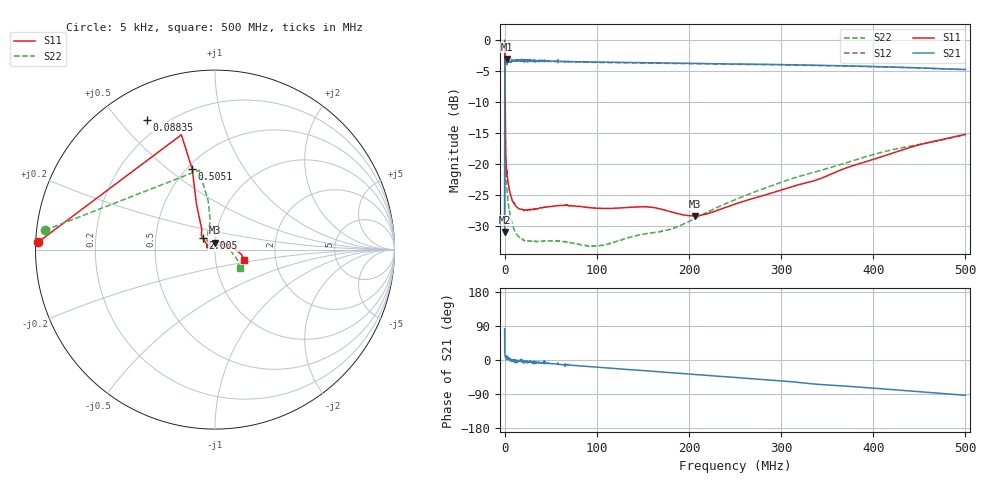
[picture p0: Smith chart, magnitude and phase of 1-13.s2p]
#  HZ  S  MA  R  50.00
! Rohde & Schwarz Vector Network Analyzer
! Rohde-Schwarz,ZNL6-2Port,1323001206101378,1.50.1.34-21.10.1.104
! Created: UTC 2/4/2024, 9:58:16 AM
! freq[Hz]  mag:S11  ang:S11  mag:S21  ang:S21  mag:S12  ang:S12  mag:S22  ang:S22
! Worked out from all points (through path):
!   6000 points, 5 kHz to 500 MHz, reference 50 ohm
!   highest |S21| = -3.12 dB at 2.505 MHz (marker M1); lowest = -30.9 dB at 5 kHz (marker M2)
!   lowest |S11| = -28.4 dB at 206.9 MHz (marker M3), VSWR 1.08, Z = 49.7 + j3.8 ohm
!   |S11| at or under -10 dB: 696.3 kHz to end of sweep
!   |S22| runs from -33.2 to -0.4 dB; largest |S21 - S12| = 0.2
!   S11 on the Smith chart (normalised r, x): 5 kHz: 0.01, +0.02; 88.35 kHz: 0.14, +0.60; 505.1 kHz: 0.53, +0.61; 2.005 MHz: 0.87, +0.11; 500 MHz: 1.38, -0.16
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5000  0.9849 177.5  0.02836 82.3  0.02766 82.9  0.9529 173.5
88346.39  0.8181 117.6  0.3065 29.1  0.3325 28.6  0.6264 112.5
505078.3  0.4646 105.8  0.5806 12.5  0.6113 7.1  0.2774 98.0
2005313  0.09171 135.8  0.6617 3.3  0.663 3.3  0.07228 130.8
2505392  0.08283 140.2  0.6983 11.1  0.6262 -5.5  0.06213 130.2
2588738  0.08196 140.4  0.6943 10.7  0.6326 -5.1  0.06095 130.3
3005470  0.0785 140.3  0.666 4.4  0.673 0.5  0.0562 131.3
3505548  0.07343 141.3  0.6625 3.2  0.6798 1.2  0.05179 132.2
4839091  0.06366 143.3  0.6658 3.6  0.6806 -1.6  0.04322 133.2
6255979  0.05717 146.0  0.6638 0.6  0.6893 -0.6  0.03789 134.8
1.04233e7  0.04897 151.3  0.6752 -4.1  0.6797 1.1  0.02956 140.7
1.550743e7  0.04367 157.5  0.6833 -1.1  0.6765 -4.5  0.02584 145.3
2.309195e7  0.04277 162.5  0.6772 -4.5  0.6788 -4.7  0.02417 148.7
4.259501e7  0.04485 164.8  0.6821 -4.1  0.6662 -13.4  0.02401 149.9
8.335139e7  0.04536 159.2  0.6638 -15.9  0.6588 -17.1  0.02233 137.0
1.052715e8  0.04389 148.1  0.6597 -19.8  0.6546 -21.4  0.02211 116.7
1.666978e8  0.04381 121.9  0.6499 -31.0  0.6451 -32.5  0.02834 73.8
2.068707e8  0.03821 92.0  0.644 -38.4  0.6401 -39.9  0.03646 41.5
2.500442e8  0.04752 61.7  0.6366 -45.9  0.6325 -48.2  0.05148 22.0
3.333906e8  0.07239 20.0  0.6214 -62.9  0.6196 -63.2  0.08476 -2.9
4.16737e8  0.1195 -2.5  0.6029 -77.3  0.6017 -77.4  0.128 -21.9
5e8  0.1731 -19.5  0.5752 -93.2  0.5742 -92.2  0.1716 -36.8
